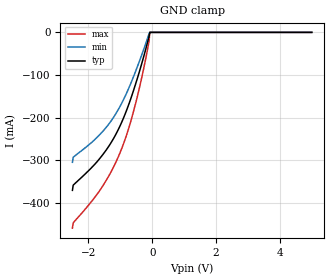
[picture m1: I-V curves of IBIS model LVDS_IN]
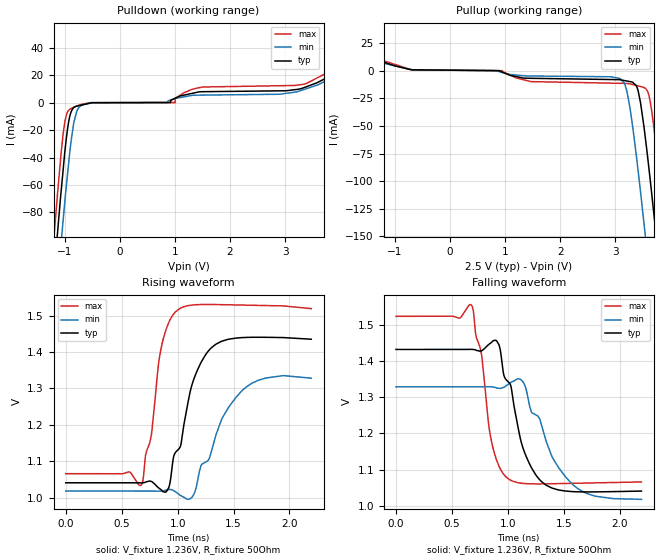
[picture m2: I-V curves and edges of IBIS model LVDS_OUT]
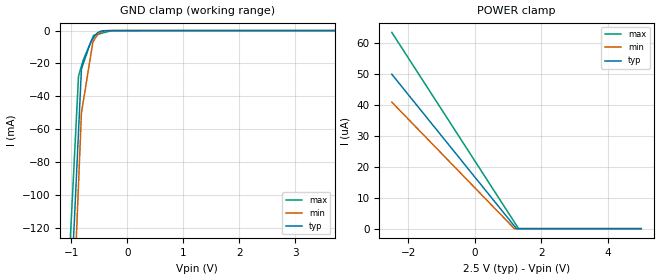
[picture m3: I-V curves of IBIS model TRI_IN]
| Texas Instruments Incorporated
| Dual 1:8 Low Additive Jitter LVDS buffer
| Marketing part#   Voltage Range   Package-type   #pins/pkg drawing
| CDCLVD2108   2.375V-3.625V   QFN   48-pin QFN
[IBIS Ver]   4.0
[File name]   cdclvd2108.ibs
[File Rev]   1.2
[Date]   10/23/2018
[Source]   spectre simulations
   Texas Instruments Incorporated.
   Analog eLab Design Center, HPA
   12500 TI Blvd
   Dallas, TX -75243
   For Support e-mail: elab_scm_ibis@list.ti.com
[Notes]   Revision History:
   Rev 1.2: 10/23/2018
   - TRI_IN model updated to reflect true electrical behavior.
   - VBB_OUT model removed  due  to inaccurary in describing
   termination behavior.
   Rev 1.1: 9/23/2013
   - Updated LVDS_IN to correct POWER and GROUND Clamp models.
   Rev 1.0: 07/06/2010
   - C_comp although listed in numberical order of value are obtained from varying PVT conditions.
   For PVT conditions for eachspecific value, refer to the buffer description under repective [Model].
   IBIS model user is responsible for using appropriate C_comp to simulate for Signal Integrity.
   - TISPice simulation of Clamp current does not match silicon
   - POWER and GND clamp for TRI_IN, D_REB_IN non-monotonic due circuit design
   - GND clamp for LVDS_IN non-monotonic due to circuit design
   - LVDS_OUT pullup/pulldown non-monotonic as a result of circuit design
[Disclaimer] This model is designed as an aid for customers of Texas Instruments.
 TI and its licensors and suppliers make no warranties, either expressed
 or implied, with respect to this  model, including the warranties of
 merchantability or fitness for a particular purpose.
 The model is provided solely on an "as is" basis. The entire risk as to
 its quality and performance is with the customer.
[Copyright] (C)Copyright 2013 Texas Instruments Incorporated.
   All rights reserved.
|   Component CDCLVD2108
[Component]   CDCLVD2108
[Manufacturer]  Texas Instruments Incorporated
[Package]   |QFN (RGZ) 48-pin
|   typ   min   max
R_pkg   0.1458   0.02281   0.16635
L_pkg   2.14842nH   0.44693nH   2.75584nH
C_pkg   0.37013pF   0.24483pF   0.72241pF
[Pin]   signal_name   model_name   R_pin   L_pin   C_pin
1   GND   GND   0.02281  0.87123n  0.72241p
2   IN_SEL   TRI_IN   0.15501  2.55939n  0.40271p
3   INP1   LVDS_IN   0.14697  2.39896n  0.38492p
4   INN1   LVDS_IN   0.14070  2.27285n  0.37078p
5   VAC_REF1   NC   0.13648  2.18679n  0.36231p
6   VCC   POWER   0.06909  1.77751n  0.40353p
7   VCC   POWER   0.13471  2.14876n  0.35406p
8   VAC_REF0   NC   0.13649  2.18683n  0.36014p
9   INN0   LVDS_IN   0.14070  2.27282n  0.37013p
10   INP0   LVDS_IN   0.14697  2.39897n  0.37485p
11   NC   NC   0.00437  0.44693n  0.24483p
12   GND   GND   0.08385  2.33255n  0.41301p
13   VCC   POWER   0.16481  2.74859n  0.38204p
14   OUTP0   LVDS_OUT   0.15475  2.55849n  0.39694p
15   OUTN0   LVDS_OUT   0.14676  2.39769n  0.38216p
16   OUTP1   LVDS_OUT   0.14055  2.27138n  0.36830p
17   OUTN1   LVDS_OUT   0.13642  2.18544n  0.35809p
18   OUTP2   LVDS_OUT   0.13475  2.14842n  0.34979p
19   OUTN2   LVDS_OUT   0.13524  2.15543n  0.35041p
20   OUTP3   LVDS_OUT   0.13790  2.20644n  0.35995p
21   OUTN3   LVDS_OUT   0.14296  2.30563n  0.37146p
22   OUTP4   LVDS_OUT   0.14998  2.44348n  0.38662p
23   OUTN4   LVDS_OUT   0.15864  2.61400n  0.40553p
24   VCC   POWER   0.08593  2.39649n  0.44857p
25   OUTP5   LVDS_OUT   0.16635  2.75577n  0.39718p
26   OUTN5   LVDS_OUT   0.15599  2.56000n  0.40575p
27   OUTP6   LVDS_OUT   0.14778  2.39690n  0.38909p
28   OUTN6   LVDS_OUT   0.14127  2.26733n  0.37409p
29   OUTP7   LVDS_OUT   0.13679  2.17708n  0.36293p
30   OUTN7   LVDS_OUT   0.13472  2.13384n  0.35313p
31   OUTP8   LVDS_OUT   0.13472  2.13391n  0.35303p
32   OUTN8   LVDS_OUT   0.13679  2.17715n  0.36285p
33   OUTP9   LVDS_OUT   0.14127  2.26735n  0.37406p
34   OUTN9   LVDS_OUT   0.14778  2.39694n  0.38905p
35   OUTP10   LVDS_OUT   0.15599  2.56007n  0.40569p
36   OUTN10   LVDS_OUT   0.16635  2.75584n  0.39710p
37   VCC   POWER   0.08575  2.38565n  0.45316p
38   OUTP11   LVDS_OUT   0.15841  2.59979n  0.41104p
39   OUTN11   LVDS_OUT   0.14979  2.43082n  0.39160p
40   OUTP12   LVDS_OUT   0.14279  2.29439n  0.37598p
41   OUTN12   LVDS_OUT   0.13775  2.19602n  0.36400p
42   OUTP13   LVDS_OUT   0.13506  2.14417n  0.35521p
43   OUTN13   LVDS_OUT   0.13457  2.13721n  0.35453p
44   OUTP14   LVDS_OUT   0.13627  2.17506n  0.36229p
45   OUTN14   LVDS_OUT   0.14038  2.26019n  0.37281p
46   OUTP15   LVDS_OUT   0.14657  2.38504n  0.38714p
47   OUTN15   LVDS_OUT   0.15452  2.54431n  0.40248p
48   VCC   POWER   0.16463  2.73633n  0.38693p
[Diff_pin]   inv_pin   vdiff   tdelay_typ   tdelay_min   tdelay_max
| The 'OUTPx' pin is Diff_pin and the 'OUTNx' pin is the inv_pin
| The 'INPX' pin is Diff_pin and the 'INNx' pin is the inv_pin
3   4   0.200   0 0 0
9   10   0.200   0 0 0
11   12   0.200   0 0 0
14   15   0.200   0 0 0
16   17   0.200   0 0 0
18   19   0.200   0 0 0
20   21   0.200   0 0 0
22   23   0.200   0 0 0
25   26   0.200   0 0 0
27   28   0.200   0 0 0
29   30   0.200   0 0 0
31   32   0.200   0 0 0
33   34   0.200   0 0 0
35   36   0.200   0 0 0
38   39   0.200   0 0 0
40   41   0.200   0 0 0
42   43   0.200   0 0 0
44   45   0.200   0 0 0
46   47   0.200   0 0 0
| Models and submodels in the file (3): LVDS_IN (Input), LVDS_OUT (Output), TRI_IN (Input)
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|   LVDS Input Model
[Model]   LVDS_IN
Model_type   Input
|Signals   INP0,INN0,INP1,INN1
Vinh = 1.6
Vinl = 0.3
| variable   typ   min   max
|   (nom PVT)   (slow PVT)   (fast PVT)
C_comp   3.121pF   2.849pF   3.193pF
| Ccomp comes from PVT, calculated at 800MHz.
| Nom PVT is nom process, 2.5V, 25C
| slow PVT is weak process, 2.375V, 105C
| Fast process is strong process, 2.625V, -40C
|   typ   min   max
[Voltage Range]   2.5   2.375   2.625
[Temperature Range]   25   105   -40
[Power Clamp Reference]   2.5   2.375   2.625
[GND Clamp Reference]   0   0   0
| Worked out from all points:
|   GND clamp passes 1 mA (typ) near -0.08 V on its own axis
[GND Clamp]
|   Voltage   I(typ)   I(min)   I(max)
-2.5V     -370.8mA   -304.9mA   -459.4mA
-2.475V   -358.5mA   -293mA     -446.8mA
-1.9V     -317.5mA   -258.4mA   -396.7mA
-1.5V     -282.1mA   -228.1mA   -354.5mA
-1.225V   -250.8mA   -200.9mA   -318mA
-975mV    -214.1mA   -169mA     -276.3mA
-700mV    -161.8mA   -124.9mA   -216.1mA
-450mV    -104.2mA   -77.57mA   -145.7mA
-150mV    -24.38mA   -14.67mA   -41.36mA
-100mV    -9.871mA   -3.55mA    -21.64mA
-75.01mV  0A         0A         0A
5V        0A         0A         0A
[POWER Clamp]
|   Voltage   I(typ)   I(min)   I(max)
-2.5V     0A         0A         0A
-2.475V   0A         0A         0A
-2.45V    0A         0A         0A
5V        0A         0A         0A
|   LVDS_OUT Model
[Model]   LVDS_OUT
Model_type   Output
| Signals   OUTP0,OUTN0,OUTP1,OUTN1,OUTP2,OUTN2,OUTP3,OUTN3,OUTP4,OUTN4,OUTP5,OUTN5,OUTP6,OUTN6
|   OUTP7,OUTN7,OUTP8,OUTN8,OUTP9,OUTN9,OUTP10,OUTN10,OUTP11,OUTN11,OUTP12,OUTN12
|   OUTP13,OUTN13,OUTP14,OUTN14,OUTP15,OUTN15
Polarity   Non-Inverting
Vmeas = 1.25
Vref = 1.25
Cref = 15pF
Rref = 50
| variable   typ   min   max
|   (nom PVT)   (slow PVT)   (fast PVT)
C_comp   1.275pF   1.175pF   1.317pF
| Ccomp comes from PVT corner simulations
| Nom PVT is nom process, 2.5V, 25C
| slow PVT is weak process, 2.375V, 105C
| Fast process is strong process, 2.625V, -40C
[Voltage Range]   2.5   2.375   2.625
[Temperature Range]   25   105   -40
[Pullup Reference]   2.5   2.375   2.625
[Pulldown Reference]   0   0   0
[Power Clamp Reference]   2.5   2.375   2.625
[GND Clamp Reference]   0   0   0
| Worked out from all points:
|   slope of the pulldown table from 0 to 0.375 V, typ, clamps not added: 11.9 kohm
|   slope of the pullup table from 0 to 0.375 V, typ, clamps not added: 2.06 kohm
|   falling waveform, V_fixture 1.236V, R_fixture 50Ohm: 20-80 % time 216ps typ, 313ps min, 114ps max; typ from 1.43 V to 1.04 V
|   rising waveform, V_fixture 1.236V, R_fixture 50Ohm: 20-80 % time 213ps typ, 297ps min, 111ps max; typ from 1.04 V to 1.44 V
[Pulldown]
|   Voltage   I(typ)   I(min)   I(max)
-2.5V     -819.9mA   -841.2mA   -808.9mA
-1.205V   -132.7mA   -170.8mA   -104.8mA
-1.179V   -119.9mA   -157.8mA   -91.4mA
-1.126V   -94.38mA   -132.6mA   -65.81mA
-1.057V   -62.54mA   -100.1mA   -34.83mA
-992.5mV  -35.05mA   -71.07mA   -13.52mA
-904.2mV  -9.792mA   -35.76mA   -4.869mA
-801.5mV  -2.839mA   -9.874mA   -2.967mA
-497.6mV  -107.4uA   -219.6uA   -77.81uA
1.006V    3.123mA    2.958mA    13.07uA
3.348V    10.9mA     9.549mA    13.39mA
4.992V    48.76mA    47.89mA    54.44mA
[Pullup]
|   Voltage   I(typ)   I(min)   I(max)
-2.5V     34.99mA    35.32mA    37.69mA
-673.6mV  752.9uA    742.8uA    631.1uA
3.09V     -8.286mA   -7.075mA   -11.46mA
3.202V    -9.311mA   -16.77mA   -11.57mA
3.31V     -10.29mA   -48.27mA   -12.56mA
3.416V    -18.21mA   -90.66mA   -13.83mA
3.525V    -51.64mA   -139.2mA   -15.42mA
3.637V    -99.27mA   -190.6mA   -28.34mA
3.71V     -133.1mA   -225.4mA   -54.42mA
3.766V    -159.3mA   -252.7mA   -79.01mA
3.928V    -237.8mA   -331.5mA   -155.2mA
4.992V    -776.9mA   -866.8mA   -698.2mA
[Ramp]
R_load = 50
|   typ   min   max
dV/dt_r   0.238696/2.15967e-10   0.19168/3.14155e-10   0.275901/1.13765e-10
dV/dt_f   0.234348/2.15967e-10   0.186163/3.14155e-10   0.274079/1.13765e-10
[Falling Waveform]
V_fixture = 1.236V
V_fixture_min = 1.173V
V_fixture_max = 1.294V
R_fixture = 50Ohm
C_fixture = 0F
|   Time   V(typ)   V(min)   V(max)
0s        1.431V     1.328V     1.523V
675ps     1.432V     1.328V     1.553V
765ps     1.428V     1.328V     1.417V
855ps     1.451V     1.328V     1.176V
920ps     1.445V     1.324V     1.11V
1.01ns    1.34V      1.337V     1.073V
1.135ns   1.16V      1.342V     1.062V
1.305ns   1.066V     1.219V     1.061V
1.62ns    1.039V     1.049V     1.062V
2.195ns   1.041V     1.018V     1.066V
[Rising Waveform]
V_fixture = 1.236V
V_fixture_min = 1.173V
V_fixture_max = 1.294V
R_fixture = 50Ohm
C_fixture = 0F
|   Time   V(typ)   V(min)   V(max)
0s        1.041V     1.018V     1.066V
675ps     1.04V      1.018V     1.035V
765ps     1.044V     1.018V     1.172V
855ps     1.021V     1.018V     1.415V
920ps     1.027V     1.022V     1.481V
1.01ns    1.133V     1.009V     1.518V
1.135ns   1.317V     1.004V     1.53V
1.305ns   1.413V     1.13V      1.531V
1.62ns    1.44V      1.306V     1.529V
2.195ns   1.435V     1.328V     1.52V
|   TRI_IN Input Model
[Model]   TRI_IN
Model_type   Input
Vinl = 0.475
Vinh = 1.8375
|   typ   min   max
C_comp   1.974pF   1.947pF   1.983pF
[Voltage Range]   2.5   2.375   2.625
[Temperature Range]   25   105   -40
[Power Clamp Reference]   2.5   2.375   2.625
[GND Clamp Reference]   0   0   0
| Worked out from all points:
|   GND clamp passes 1 mA (typ) near -0.51 V on its own axis
[GND Clamp]
|   Voltage   I(typ)   I(min)   I(max)
-2.5V     -1.519A    -1.599A    -1.46A
-1.383V   -435.2mA   -519.8mA   -372mA
-872mV    -61.4mA    -93.54mA   -27.86mA
-820mV    -23.3mA    -50.1mA    -21.6mA
-782.5mV  -19.62mA   -42.18mA   -17.41mA
-670mV    -8.564mA   -18.42mA   -8.334mA
-617.5mV  -5.055mA   -7.338mA   -4.098mA
-602.5mV  -4.217mA   -6.329mA   -2.888mA
-497.5mV  -686.1uA   -1.614mA   -1.968mA
-415mV    -96.99uA   -336uA     -1.246mA
-275.7mV  -21.08uA   -26.56uA   -26.45uA
5V        0A         0A         0A
[POWER Clamp]
|   Voltage   I(typ)   I(min)   I(max)
-2.5V     49.93uA    40.92uA    63.45uA
1.183V    882.3nA    41.92nA    2.147uA
1.242V    83.42nA    0A         1.149uA
1.31V     0A         0A         25.11nA
5V        0A         0A         0A
